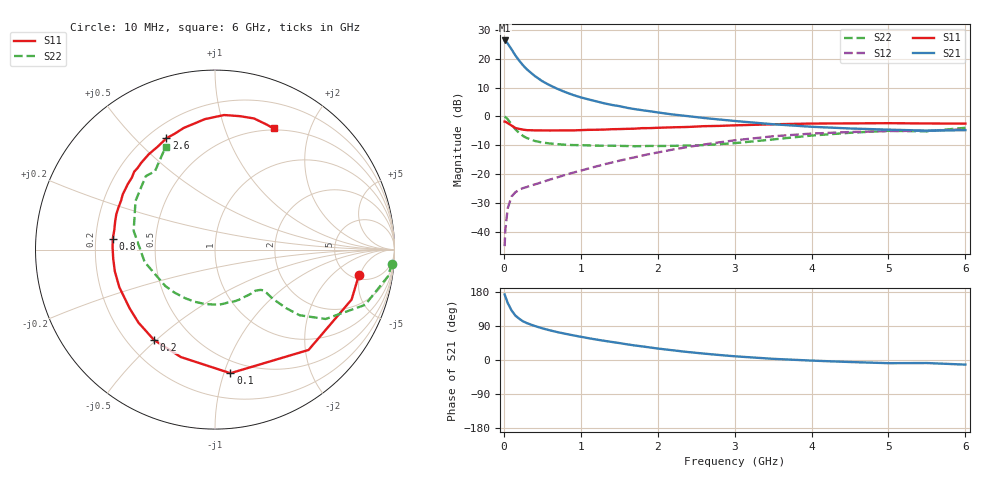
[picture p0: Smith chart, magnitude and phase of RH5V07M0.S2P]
! SIEMENS Small Signal Semiconductors
! BFR106
! Si NPN RF Bipolar Junction Transistor in SOT23
! VCE = 5 V  IC = 7 mA
! Common Emitter S-Parameters:  August  1996
# GHz  S  MA  R  50
!  f  S11  S21  S12  S22
! GHz  MAG  ANG  MAG  ANG  MAG  ANG  MAG  ANG
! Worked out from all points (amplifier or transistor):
!   36 points, 10 MHz to 6 GHz, reference 50 ohm
!   highest |S21| = 26.4 dB at 10 MHz (marker M1)
!   |S21| within 3 dB of that: start of sweep to 98.57 MHz
!   unconditionally stable (mu >= 1): 557.1 MHz to 1.951 GHz; 5.088 GHz to end of sweep
!   at 250 MHz: K = 0.60, MSG = 21.3 dB, |S12| = -24.9 dB
!   at 1.4 GHz: K = 1.12, MAG = 7.9 dB, |S12| = -16.0 dB
!   at 6 GHz: K = 1.02, MAG = -0.9 dB, |S12| = -4.5 dB
!   S11 on the Smith chart (normalised r, x): 10 MHz: 5.64, -4.78; 100 MHz: 0.40, -1.05; 200 MHz: 0.31, -0.49; 800 MHz: 0.27, +0.05; 2.6 GHz: 0.27, +0.62; 6 GHz: 0.48, +1.48
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0.01  0.8141 -10.1  20.79 173.0  0.0056 85.8  0.9891 -4.5
0.02  0.8103 -20.1  20.59 167.6  0.0109 81.2  0.9753 -8.8
0.05  0.7644 -47.0  18.4 150.6  0.0253 67.7  0.8914 -20.2
0.1  0.694 -82.9  14.62 131.0  0.0407 54.1  0.7276 -32.1
0.15  0.6282 -107.6  11.43 117.2  0.0483 46.2  0.5968 -37.8
0.2  0.6076 -124.0  9.277 108.9  0.0533 44.0  0.5163 -39.4
0.25  0.5893 -136.4  7.686 102.0  0.057 42.8  0.4568 -40.0
0.3  0.5774 -145.4  6.548 97.3  0.0597 43.8  0.4211 -40.4
0.4  0.5728 -158.5  5.053 89.9  0.0659 45.6  0.3754 -40.0
0.5  0.5711 -167.8  4.079 83.6  0.0725 48.3  0.352 -40.2
0.6  0.5694 -174.8  3.453 78.2  0.0801 51.4  0.3387 -41.5
0.8  0.5727 174.0  2.635 69.2  0.0966 55.9  0.3217 -45.4
0.9  0.5715 169.1  2.354 65.1  0.1057 57.9  0.318 -47.5
1.1  0.5842 160.2  1.972 57.6  0.1247 60.5  0.3141 -54.0
1.3  0.5901 152.5  1.692 50.8  0.1468 61.9  0.3094 -60.6
1.6  0.608 142.9  1.411 41.4  0.1827 62.4  0.3059 -72.4
2.2  0.6467 124.9  1.078 25.5  0.2661 58.4  0.3082 -100.0
2.6  0.6766 113.6  0.939 16.9  0.3249 53.2  0.3178 -121.6
3.5  0.7292 94.4  0.731 3.1  0.4519 38.0  0.3981 -170.0
4.5  0.7564 79.4  0.617 -5.3  0.5355 19.2  0.5193 148.5
5.5  0.7539 67.7  0.566 -8.0  0.5641 7.0  0.5499 127.5
6  0.7497 64.2  0.577 -12.2  0.5967 -1.0  0.6348 115.7
